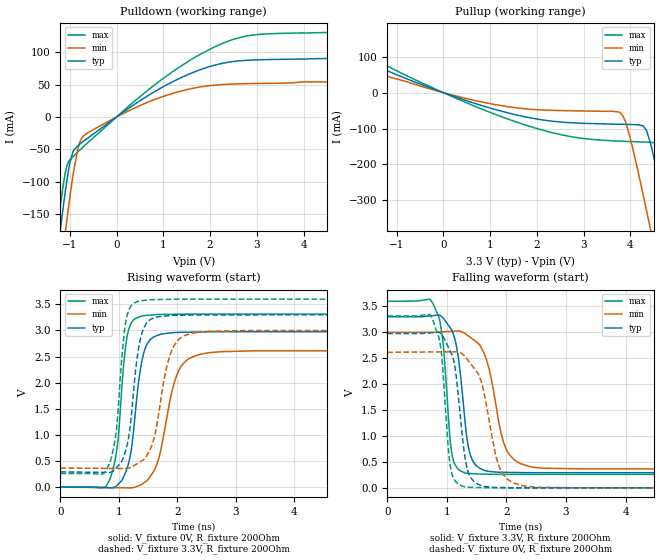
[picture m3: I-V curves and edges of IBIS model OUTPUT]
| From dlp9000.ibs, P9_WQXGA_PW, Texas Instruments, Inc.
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|   Model
[Model]   OUTPUT
Model_type   Output
Polarity   Non-Inverting
Vmeas = 1.65
Vref = 0
Cref = 1pF
Rref = 100000
|   typ   min   max
C_comp   1.893pF   1.813pF   2.012pF
[Voltage Range]   3.3   3   3.6
[Temperature Range]   25   125   -40
[Pullup Reference]   3.3   3   3.6
[Pulldown Reference]   -0   -0   -0
[Power Clamp Reference]   3.3   3   3.6
[GND Clamp Reference]   -0   -0   -0
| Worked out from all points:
|   slope of the pulldown table from 0 to 0.495 V, typ, clamps not added: 19.9 ohm
|   slope of the pullup table from 0 to 0.495 V, typ, clamps not added: 22.1 ohm
|   falling waveform, V_fixture 3.3V, R_fixture 200Ohm: 20-80 % time 179ps typ, 284ps min, 133ps max; typ from 3.3 V to 0.292 V
|   rising waveform, V_fixture 0V, R_fixture 200Ohm: 20-80 % time 195ps typ, 299ps min, 153ps max; typ from 0 V to 2.98 V
|   rising waveform, V_fixture 3.3V, R_fixture 200Ohm: 20-80 % time 188ps typ, 272ps min, 152ps max; typ from 0.292 V to 3.3 V
|   falling waveform, V_fixture 0V, R_fixture 200Ohm: 20-80 % time 175ps typ, 280ps min, 129ps max; typ from 2.98 V to 0 V
[Pulldown]
|   Voltage   I(typ)   I(min)   I(max)
-3.3V     -1.529A    -1.592A    -1.493A
-1.261V   -208.9mA   -275.8mA   -170.2mA
-1.191V   -168mA     -234mA     -131mA
-1.102V   -118.5mA   -181.7mA   -88.26mA
-1.063V   -98.4mA    -159.1mA   -75.77mA
-933.9mV  -54.1mA    -91.29mA   -61.3mA
-825mV    -44.19mA   -48.2mA    -53.68mA
-686.4mV  -36.38mA   -27.93mA   -44.24mA
858mV     41.07mA    28.19mA    52.01mA
2.224V    82.41mA    50mA       112.5mA
3.056V    88.48mA    51.91mA    127.7mA
6.59V     97.93mA    59.65mA    138.4mA
[Pullup]
|   Voltage   I(typ)   I(min)   I(max)
-3.3V     147.3mA    116.3mA    179.2mA
1.393V    -56.71mA   -39.35mA   -74.21mA
2.64V     -83.17mA   -50.31mA   -120.6mA
3.759V    -88.14mA   -54.33mA   -135.2mA
3.887V    -88.47mA   -78.64mA   -135.9mA
3.996V    -88.77mA   -126.8mA   -136.5mA
4.274V    -92.63mA   -285mA     -137.7mA
4.432V    -142.3mA   -382.4mA   -138.7mA
4.729V    -314.5mA   -570mA     -143.6mA
4.828V    -376.3mA   -633.3mA   -167.4mA
5.214V    -622.8mA   -882.4mA   -392.9mA
6.59V     -1.523A    -1.783A    -1.29A
[Ramp]
R_load = 200
|   typ   min   max
dV/dt_r   1.7857/1.94071e-10   1.56877/2.98371e-10   1.9883/1.52481e-10
dV/dt_f   1.80494/1.7937e-10   1.58128/2.84231e-10   2.00394/1.329e-10
[Falling Waveform]
V_fixture = 3.3V
V_fixture_min = 3V
V_fixture_max = 3.6V
R_fixture = 200Ohm
C_fixture = 0F
|   Time   V(typ)   V(min)   V(max)
0s        3.3V       3V         3.6V
784.7ps   3.323V     3.001V     3.51V
934.7ps   3.279V     3.011V     2.81V
1.092ns   3.017V     3.02V      613.2mV
1.297ns   1.371V     2.982V     290.1mV
1.499ns   422.2mV    2.812V     267.8mV
1.708ns   317.2mV    2.3V       262.7mV
1.984ns   299.6mV    777.8mV    260.4mV
2.4ns     292.2mV    407.9mV    260.3mV
10ns      291.7mV    364.5mV    260.1mV
[Rising Waveform]
V_fixture = 0V
V_fixture_min = 0V
V_fixture_max = 0V
R_fixture = 200Ohm
C_fixture = 0F
|   Time   V(typ)   V(min)   V(max)
0s        16.17uV    35.15uV    916.2nV
834.4ps   -12.26mV   -9.994mV   121.3mV
976.5ps   39.27mV    -11.7mV    806.9mV
1.144ns   373.1mV    -13.72mV   2.9V
1.219ns   756.6mV    -14.35mV   3.156V
1.375ns   2.286V     42.53mV    3.271V
1.685ns   2.915V     553.2mV    3.306V
2.019ns   2.963V     2.22V      3.311V
2.4ns     2.971V     2.546V     3.313V
10ns      2.976V     2.615V     3.314V
[Rising Waveform]
V_fixture = 3.3V
V_fixture_min = 3V
V_fixture_max = 3.6V
R_fixture = 200Ohm
C_fixture = 0F
|   Time   V(typ)   V(min)   V(max)
0s        291.7mV    364.5mV    260.1mV
827.1ps   280.8mV    357.7mV    420.1mV
956.3ps   367.4mV    356.6mV    1.079V
1.065ns   535.1mV    355.7mV    2.667V
1.147ns   829.7mV    359.3mV    3.304V
1.321ns   2.532V     453.5mV    3.554V
1.577ns   3.228V     839.5mV    3.59V
1.915ns   3.289V     2.641V     3.597V
2.237ns   3.295V     2.942V     3.599V
10ns      3.3V       3V         3.6V
[Falling Waveform]
|Gnd
V_fixture = 0V
V_fixture_min = 0V
V_fixture_max = 0V
R_fixture = 200Ohm
C_fixture = 0F
|   Time   V(typ)   V(min)   V(max)
0s        2.976V     2.615V     3.314V
757.8ps   2.991V     2.621V     3.257V
904.2ps   2.966V     2.622V     2.639V
1.065ns   2.615V     2.623V     369.3mV
1.147ns   2.248V     2.624V     122.1mV
1.262ns   972.3mV    2.578V     31.24mV
1.45ns    126mV      2.317V     8.353mV
1.887ns   7.381mV    385.2mV    465.9uV
2.237ns   937.8uV    51.02mV    445.8uV
10ns      16.18uV    35.48uV    916.2nV
